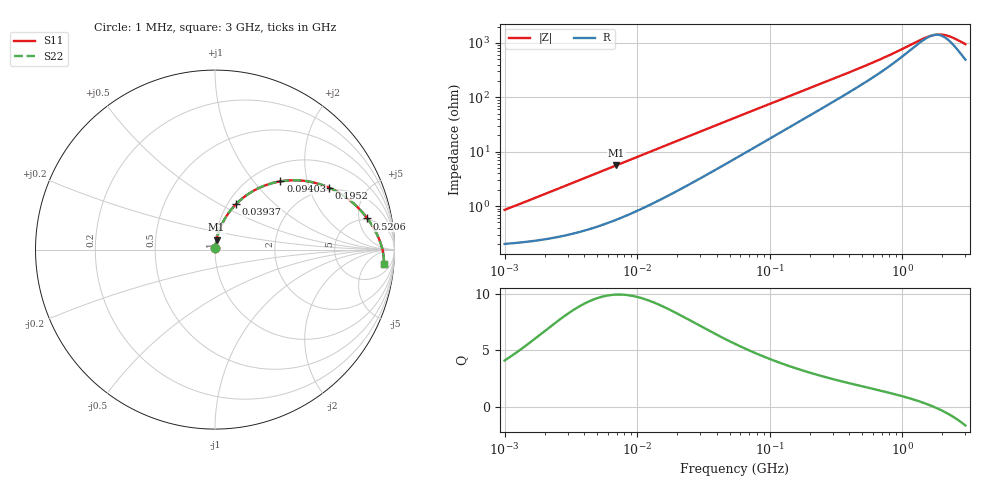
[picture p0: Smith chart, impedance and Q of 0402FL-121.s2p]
# MHz S MA R 50
!Freq  MagS11  AngS11  MagS21  AngS21  MagS12  AngS12  MagS22  AngS22
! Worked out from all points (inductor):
!   801 points, 1 MHz to 3 GHz, reference 50 ohm
!   read as one part in series: L = 131 nH near 1.041 MHz
!   highest Q = 9.95 at 6.97 MHz (marker M1), where L = 127 nH
!   self-resonance near 1.732 GHz
!   S11 on the Smith chart (normalised r, x): 1 MHz: 1.00, +0.02; 39.37 MHz: 1.09, +0.60; 94.03 MHz: 1.32, +1.39; 195.2 MHz: 1.89, +2.73; 520.6 MHz: 4.70, +6.54; 3 GHz: 11, -16
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1  0.008496 75.8  0.998 -0.5  0.998 -0.5  0.008496 75.8
3.823119  0.03102 81.9  0.9961 -1.8  0.9961 -1.8  0.03102 81.9
6.969505  0.05569 81.1  0.9929 -3.2  0.9929 -3.2  0.05569 81.1
14.47069  0.1127 77.3  0.9814 -6.4  0.9814 -6.4  0.1127 77.3
25.09235  0.1885 71.8  0.958 -10.8  0.958 -10.8  0.1885 71.8
39.36673  0.2803 65.1  0.9178 -16.1  0.9178 -16.1  0.2803 65.1
54.77226  0.3658 58.7  0.8684 -21.1  0.8684 -21.1  0.3658 58.7
71.05049  0.4416 53.0  0.8143 -25.7  0.8143 -25.7  0.4416 53.0
94.02997  0.5268 46.2  0.7406 -30.9  0.7406 -30.9  0.5268 46.2
133.4721  0.6289 37.5  0.6306 -37.4  0.6306 -37.4  0.6289 37.5
195.2332  0.7228 28.6  0.5026 -43.4  0.5026 -43.4  0.7228 28.6
209.4008  0.7376 27.0  0.4795 -44.3  0.4795 -44.3  0.7376 27.0
325.2521  0.813 18.5  0.3453 -48.4  0.3453 -48.4  0.813 18.5
520.5962  0.8661 11.6  0.2307 -48.9  0.2307 -48.9  0.8661 11.6
792.5923  0.8976 6.9  0.1528 -44.6  0.1528 -44.6  0.8976 6.9
1444.887  0.9268 1.5  0.07738 -18.3  0.07738 -18.3  0.9268 1.5
1613.037  0.9307 0.6  0.06997 -7.8  0.06997 -7.8  0.9307 0.6
1782.824  0.9339 -0.2  0.06619 3.4  0.06619 3.4  0.9339 -0.2
1970.482  0.9368 -1.1  0.06579 15.6  0.06579 15.6  0.9368 -1.1
2199.798  0.9396 -2.0  0.06947 28.5  0.06947 28.5  0.9396 -2.0
2455.801  0.9419 -3.0  0.07718 39.7  0.07718 39.7  0.9419 -3.0
3000  0.9449 -4.9  0.09948 53.9  0.09948 53.9  0.9449 -4.9
